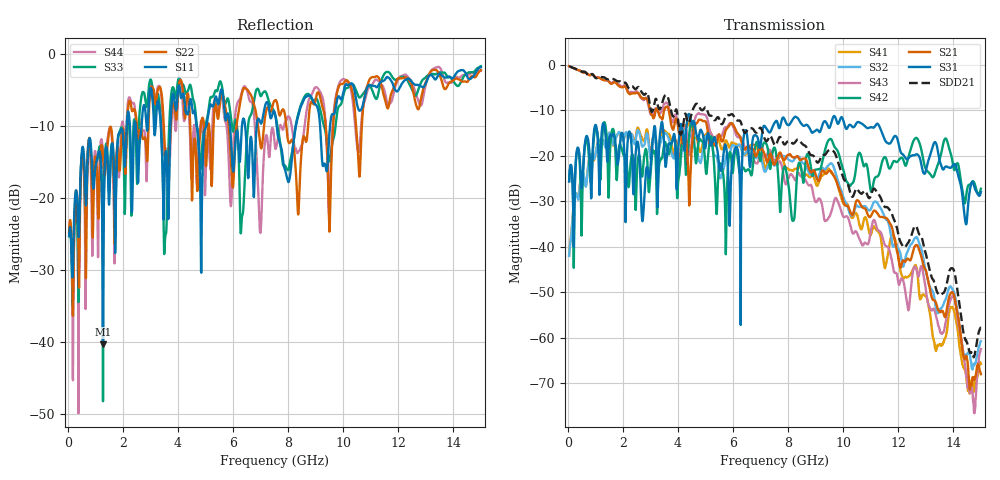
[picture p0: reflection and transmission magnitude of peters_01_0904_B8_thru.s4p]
# MHZ S RI R 50.00
! FREQ  S11  S12  S13  S14
!  S21  S22  S23  S24
!  S31  S32  S33  S34
!  S41  S42  S43  S44
!  REAL  IMAG  REAL  IMAG  REAL  IMAG  REAL  IMAG
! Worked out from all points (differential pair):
!   1496 points, 50 MHz to 15 GHz, reference 50 ohm
!   strongest paths, dB at 50 MHz, 3.79 GHz, 7.53 GHz, 11.27 GHz, 15 GHz:
!     S31: -25.6, -17.0, -12.6, -13.1, -28.0
!     S21: -0.3, -13.9, -21.6, -32.9, -68.0
!     S42: -25.6, -17.0, -18.5, -24.4, -27.2
!     S43: -0.3, -12.5, -21.5, -36.3, -62.4
!     S32: -42.0, -20.0, -22.0, -30.7, -60.7
!     S41: -41.9, -18.5, -21.3, -36.7, -65.7
!   taken as a pair (ports 1,3 in; 2,4 out), SDD21 dB: -0.3, -10.9, -17.7, -28.3, -57.8
!   lowest |S11| = -40.3 dB at 1.28 GHz (marker M1), VSWR 1.02, Z = 50.6 - j0.745 ohm
!   |S11| at or under -10 dB: start of sweep to 2.142 GHz; 5.89 GHz to 6.327 GHz (436.9 MHz wide, 7.15 % of centre); 7.587 GHz to 8.286 GHz (699 MHz wide, 8.81 % of centre)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
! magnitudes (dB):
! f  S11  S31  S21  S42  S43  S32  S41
! 50 MHz  -25.3  -25.6  -0.3  -25.6  -0.3  -42.0  -41.9
! 1.28 GHz  -40.3  -12.9  -3.4  -14.0  -3.3  -16.5  -16.7
! 2.72 GHz  -8.1  -34.3  -7.3  -24.0  -7.6  -18.0  -16.4
! 3.54 GHz  -14.3  -21.8  -9.5  -17.0  -8.5  -15.1  -14.7
! 4.05 GHz  -4.5  -15.5  -15.4  -24.1  -14.6  -23.2  -21.3
! 9.48 GHz  -12.2  -13.9  -23.3  -16.5  -33.6  -22.0  -22.9
! 15 GHz  -1.9  -28.0  -68.0  -27.2  -62.4  -60.7  -65.7
